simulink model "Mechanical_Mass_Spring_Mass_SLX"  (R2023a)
settings: Solver=ode23s  StartTime=0.0  StopTime=10.0  MaxStep=0.001  RelTol=1e-3
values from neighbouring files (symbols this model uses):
  b_3 = 2*N/(m/sec)    (= 2)    [Mechanical_Mass_Spring_Mass_EQN.m]    (also in Mechanical_Mass_Spring_Mass_SLX_m.m; Car_Dumper_EQN.m; Car_Dumper_SLX_m.m; Mechanical_Transmission_EQN.m)
  b_6 = 2*N/(m/sec)    (= 2)    [Mechanical_Mass_Spring_Mass_EQN.m]    (also in Mechanical_Mass_Spring_Mass_SLX_m.m; Car_Dumper_EQN.m; Car_Dumper_SLX_m.m; Mechanical_Transmission_EQN.m)
  b_7 = 2*N/(m/sec)    (= 2)    [Mechanical_Mass_Spring_Mass_EQN.m]    (also in Mechanical_Mass_Spring_Mass_SLX_m.m; Car_Dumper_EQN.m; Car_Dumper_SLX_m.m; Electrical_DC_Motor_EQN.m = 0.1)
  F_1_0 = 10*N    (= 10)    [Mechanical_Mass_Spring_Mass_SLX_m.m]    (also in Car_Dumper_SLX_m.m; Mechanical_Transmission_SLX_m.m)
  F_4_0 = 0*N    (= 0)    [Mechanical_Mass_Spring_Mass_SLX_m.m]    (also in Car_Dumper_SLX_m.m; Mechanical_Transmission_SLX_m.m)
  K_4 = 1000*N/m    (= 1000)    [Mechanical_Mass_Spring_Mass_EQN.m]    (also in Mechanical_Mass_Spring_Mass_SLX_m.m; Car_Dumper_EQN.m; Car_Dumper_SLX_m.m; Mechanical_Transmission_EQN.m)
  M_2 = 0.5*kg    (= 0.5)    [Mechanical_Mass_Spring_Mass_EQN.m]    (also in Mechanical_Mass_Spring_Mass_SLX_m.m; Car_Dumper_EQN.m; Car_Dumper_SLX_m.m; Mechanical_Transmission_EQN.m)
  M_5 = 0.5*kg    (= 0.5)    [Mechanical_Mass_Spring_Mass_EQN.m]    (also in Mechanical_Mass_Spring_Mass_SLX_m.m; Car_Dumper_EQN.m; Car_Dumper_SLX_m.m; Mechanical_Transmission_EQN.m)
  Ts = Tfin/Nr_Ts_Points    (= 0.001001)    [Mechanical_Mass_Spring_Mass_SLX_m.m]    (also in BIG_EC_Simscape_SLX_m.m = 0.0003; Car_Dumper_SLX_m.m = 0.0022779; Electric_Circuit_01_SLX_m.m = 0.005; Electric_Circuit_02_SLX_m.m = 0.000480145)
  v_2_0 = 0*m/sec    (= 0)    [Mechanical_Mass_Spring_Mass_SLX_m.m]    (also in Car_Dumper_SLX_m.m; Mechanical_Transmission_SLX_m.m)
  v_5_0 = 0*m/sec    (= 0)    [Mechanical_Mass_Spring_Mass_SLX_m.m]    (also in Car_Dumper_SLX_m.m; Mechanical_Transmission_SLX_m.m)
  v_8_0 = 0*m/sec    (= 0)    [Mechanical_Mass_Spring_Mass_SLX_m.m]

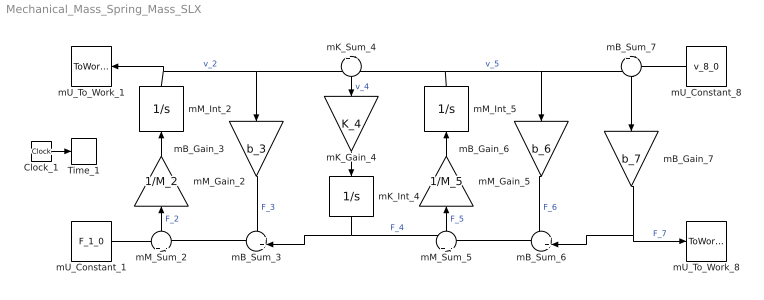
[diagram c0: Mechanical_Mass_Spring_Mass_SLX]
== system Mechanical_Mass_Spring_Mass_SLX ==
  Clock_1 : Clock
  Time_1 : ToWorkspace  VariableName=t  SaveFormat=Timeseries  SampleTime=Ts
  mB_Gain_3 : Gain  Gain=b_3  Multiplication=Matrix(K*u)
  mB_Gain_6 : Gain  Gain=b_6  Multiplication=Matrix(K*u)
  mB_Gain_7 : Gain  Gain=b_7  Multiplication=Matrix(K*u)
  mB_Sum_3 : Sum  Inputs=++|
  mB_Sum_6 : Sum  Inputs=++|
  mB_Sum_7 : Sum  Inputs=+|-
  mK_Gain_4 : Gain  Gain=K_4  Multiplication=Matrix(K*u)
  mK_Int_4 : Integrator  InitialCondition=F_4_0
  mK_Sum_4 : Sum  Inputs=+|-
  mM_Gain_2 : Gain  Gain=1/M_2  Multiplication=Matrix(K*u)
  mM_Gain_5 : Gain  Gain=1/M_5  Multiplication=Matrix(K*u)
  mM_Int_2 : Integrator  InitialCondition=v_2_0
  mM_Int_5 : Integrator  InitialCondition=v_5_0
  mM_Sum_2 : Sum  Inputs=+|-
  mM_Sum_5 : Sum  Inputs=+|-
  mU_Constant_1 : Constant  Value=F_1_0
  mU_Constant_8 : Constant  Value=v_8_0
  mU_To_Work_1 : ToWorkspace  VariableName=v_1_0  SaveFormat=Timeseries  SampleTime=Ts
  mU_To_Work_8 : ToWorkspace  VariableName=F_8_0  SaveFormat=Timeseries  SampleTime=Ts
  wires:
  mU_Constant_1/1 -> mM_Sum_2/1
  mB_Sum_3/1 -> mM_Sum_2/2
  mM_Int_2/1 -> mU_To_Work_1/1, mB_Gain_3/1, mK_Sum_4/1  "v_2"
  mM_Sum_2/1 -> mM_Gain_2/1  "F_2"
  mM_Gain_2/1 -> mM_Int_2/1
  mK_Int_4/1 -> mB_Sum_3/2, mM_Sum_5/1  "F_4"
  mB_Gain_3/1 -> mB_Sum_3/1  "F_3"
  mM_Int_5/1 -> mK_Sum_4/2, mB_Gain_6/1, mB_Sum_7/1  "v_5"
  mK_Sum_4/1 -> mK_Gain_4/1  "v_4"
  mK_Gain_4/1 -> mK_Int_4/1
  mB_Sum_6/1 -> mM_Sum_5/2
  mM_Sum_5/1 -> mM_Gain_5/1  "F_5"
  mM_Gain_5/1 -> mM_Int_5/1
  mB_Gain_7/1 -> mB_Sum_6/2, mU_To_Work_8/1  "F_7"
  mB_Gain_6/1 -> mB_Sum_6/1  "F_6"
  mU_Constant_8/1 -> mB_Sum_7/2
  mB_Sum_7/1 -> mB_Gain_7/1
  Clock_1/1 -> Time_1/1
